| TEXAS INSTRUMENTS INCORPORATED
| Standard Linear and Logic Group
| IBIS Model of SN74ALVCH162827
| 20-BIT BUFFER/DRIVER WITH 3-STATE OUTPUTS
| This file contains package information for the following:
|  TSSOP 56-pin (DGG) package as [Component] ALVCH162827_DGG
|  TVSOP 56-pin (DGV) package as [Component] ALVCH162827_DGV
|  SSOP 56-pin (DL) package as [Component] ALVCH162827_DL
| This device can be powered at the following Vccs:
|  1.8 volt Vcc
|  2.5 volt Vcc
|  2.7 volt Vcc
|  3.3 volt Vcc
| This file provides unique models under the [Model Selector] for each Vcc.
| For operation at a specific Vcc, select the appropriate model after each
| [Model Selector] keyword.
[IBIS Ver]   3.2
[Comment char]  |_char
[File Name]   sn74alvch162827.ibs
[File Rev]   1.1 | a_die
[Date]   May 5, 2003
[Source]   Data created from TI-SPICE simulations at TI-SLL.
[Notes]   The following is an IBIS list for the ALVCH162827.
   Please contact sllibis@ti.com with questions and
   comments concerning SLL IBIS models.
   This IBIS model is created from a BA (back annotated
   netlist)
   - Non-monotonic data in ground-clamp due to bus-hold
[Disclaimer] Property of Texas Instruments Incorporated.  Unauthorized
   reproduction and/or distribution is strictly prohibited.
   This product is protected under copyright law.
   Created  2003, (C) Copyright  2003, Texas Instruments
   Incorporated, All Rights Reserved
   UNLESS THERE IS A SIGNED, WRITTEN AGREEMENT TO THE
   CONTRARY, TEXAS INSTRUMENTS (TI) IS PROVIDING THE IBIS
   MODELS  AND WITHOUT ANY WARRANTY, EXPRESSED OR
   IMPLIED.  TI assumes no liability for:
   1) the accuracy of the IBIS models provided to your
   company;
   2) the proper functioning of these IBIS Models in your
   design or for any resulting applications; or
   3) infringement of patents, copyrights or intellectual
   property rights resulting from your use of these IBIS
   models.
   TI provides IBIS Models as a service to our customers.
   You and your company shall not distribute, sell or give
   these models to anyone else without prior written
   permission from TI.
   TI reserves the right to make changes to our products or
   to discontinue any semiconductor product or service
   without notice, and advises our customers to obtain the
   latest version of relevant information to verify, before
   placing orders, that the information being relied on is
   current.
   Please be aware that your receipt and use of the IBIS
   information provided shall serve as acceptance of these
   terms and conditions.  If you do not accept these terms,
   you should return or destroy the IBIS models and any
   other accompanying information immediately.
| Component ALVCH162827_DGG 56-pin TSSOP
[Component]   ALVCH162827_DGG
[Manufacturer]   Texas Instruments, Inc.
[Package]
|   typ   min   max
R_pkg   4.500e-02   3.500e-02   6.200e-02
L_pkg   3.324e-09   2.403e-09   5.094e-09
C_pkg   5.640e-13   3.410e-13   9.140e-13
[Pin]   signal_name   model_name   R_pin   L_pin   C_pin
1   1NOE1   ALVCH162827_OE   6.200e-02   5.094e-09   8.560e-13
2   1Y1   ALVCH162827_OUT   6.100e-02   4.621e-09   9.020e-13
3   1Y2   ALVCH162827_OUT   6.000e-02   4.316e-09   8.020e-13
4   GND   GND   5.900e-02   3.968e-09   6.980e-13
5   1Y3   ALVCH162827_OUT   5.700e-02   3.716e-09   6.490e-13
6   1Y4   ALVCH162827_OUT   4.200e-02   3.517e-09   6.530e-13
7   VCC   POWER   4.100e-02   3.160e-09   5.700e-13
8   1Y5   ALVCH162827_OUT   3.900e-02   2.981e-09   4.820e-13
9   1Y6   ALVCH162827_OUT   3.900e-02   2.808e-09   4.470e-13
10   1Y7   ALVCH162827_OUT   3.800e-02   2.715e-09   4.090e-13
11   GND   GND   4.100e-02   2.675e-09   3.910e-13
12   1Y8   ALVCH162827_OUT   3.900e-02   2.536e-09   3.660e-13
13   1Y9   ALVCH162827_OUT   3.900e-02   2.457e-09   3.480e-13
14   1Y10   ALVCH162827_OUT   3.800e-02   2.411e-09   3.530e-13
15   2Y1   ALVCH162827_OUT   3.900e-02   2.456e-09   3.550e-13
16   2Y2   ALVCH162827_OUT   3.900e-02   2.471e-09   3.490e-13
17   2Y3   ALVCH162827_OUT   4.000e-02   2.580e-09   3.700e-13
18   GND   GND   3.800e-02   2.651e-09   3.890e-13
19   2Y4   ALVCH162827_OUT   3.800e-02   2.739e-09   4.110e-13
20   2Y5   ALVCH162827_OUT   3.900e-02   2.838e-09   4.490e-13
21   2Y6   ALVCH162827_OUT   3.800e-02   2.988e-09   4.840e-13
22   VCC   POWER   3.800e-02   3.104e-09   5.640e-13
23   2Y7   ALVCH162827_OUT   4.000e-02   3.427e-09   6.380e-13
24   2Y8   ALVCH162827_OUT   5.600e-02   3.654e-09   6.410e-13
25   GND   GND   5.700e-02   3.932e-09   7.000e-13
26   2Y9   ALVCH162827_OUT   5.800e-02   4.257e-09   8.060e-13
27   2Y10   ALVCH162827_OUT   5.700e-02   4.580e-09   9.140e-13
28   2NOE1   ALVCH162827_OE   5.900e-02   5.038e-09   8.610e-13
29   2NOE2   ALVCH162827_OE   6.000e-02   5.058e-09   8.580e-13
30   2A10   ALVCH162827_IN   5.600e-02   4.543e-09   9.040e-13
31   2A9   ALVCH162827_IN   5.700e-02   4.241e-09   8.020e-13
32   GND   GND   5.900e-02   3.933e-09   6.990e-13
33   2A8   ALVCH162827_IN   5.600e-02   3.616e-09   6.370e-13
34   2A7   ALVCH162827_IN   3.700e-02   3.368e-09   6.400e-13
35   VCC   POWER   3.600e-02   3.024e-09   5.630e-13
36   2A6   ALVCH162827_IN   3.500e-02   2.876e-09   4.740e-13
37   2A5   ALVCH162827_IN   3.500e-02   2.745e-09   4.440e-13
38   2A4   ALVCH162827_IN   3.700e-02   2.683e-09   4.050e-13
39   GND   GND   3.800e-02   2.603e-09   3.820e-13
40   2A3   ALVCH162827_IN   3.800e-02   2.510e-09   3.620e-13
41   2A2   ALVCH162827_IN   3.600e-02   2.412e-09   3.410e-13
42   2A1   ALVCH162827_IN   3.800e-02   2.416e-09   3.490e-13
43   1A10   ALVCH162827_IN   3.800e-02   2.403e-09   3.490e-13
44   1A9   ALVCH162827_IN   3.700e-02   2.429e-09   3.410e-13
45   1A8   ALVCH162827_IN   3.600e-02   2.483e-09   3.580e-13
46   GND   GND   3.700e-02   2.614e-09   3.810e-13
47   1A7   ALVCH162827_IN   3.500e-02   2.669e-09   4.020e-13
48   1A6   ALVCH162827_IN   3.600e-02   2.763e-09   4.420e-13
49   1A5   ALVCH162827_IN   3.600e-02   2.942e-09   4.780e-13
50   VCC   POWER   3.500e-02   3.053e-09   5.640e-13
51   1A4   ALVCH162827_IN   3.600e-02   3.408e-09   6.410e-13
52   1A3   ALVCH162827_IN   5.800e-02   3.698e-09   6.410e-13
53   GND   GND   5.900e-02   3.974e-09   6.970e-13
54   1A2   ALVCH162827_IN   6.100e-02   4.327e-09   8.020e-13
55   1A1   ALVCH162827_IN   6.100e-02   4.624e-09   9.050e-13
56   1NOE2   ALVCH162827_OE   6.000e-02   5.063e-09   8.580e-13
| Component ALVCH162827_DGV 56-pin TVSOP
[Component]   ALVCH162827_DGV
[Manufacturer]   Texas Instruments, Inc.
[Package]
|   typ   min   max
R_pkg   6.300e-02   5.000e-02   8.400e-02
L_pkg   2.945e-09   2.394e-09   3.939e-09
C_pkg   3.910e-13   2.710e-13   5.880e-13
[Pin]   signal_name   model_name   R_pin   L_pin   C_pin
1   1NOE1   ALVCH162827_OE   6.800e-02   3.933e-09   5.880e-13
2   1Y1   ALVCH162827_OUT   6.800e-02   3.568e-09   5.870e-13
3   1Y2   ALVCH162827_OUT   7.600e-02   3.464e-09   5.150e-13
4   GND   GND   8.400e-02   3.444e-09   4.590e-13
5   1Y3   ALVCH162827_OUT   8.100e-02   3.277e-09   4.270e-13
6   1Y4   ALVCH162827_OUT   7.400e-02   3.136e-09   3.870e-13
7   VCC   POWER   6.900e-02   2.970e-09   4.010e-13
8   1Y5   ALVCH162827_OUT   5.000e-02   2.785e-09   3.790e-13
9   1Y6   ALVCH162827_OUT   5.100e-02   2.685e-09   3.200e-13
10   1Y7   ALVCH162827_OUT   5.300e-02   2.611e-09   3.160e-13
11   GND   GND   5.300e-02   2.495e-09   2.970e-13
12   1Y8   ALVCH162827_OUT   5.300e-02   2.435e-09   2.920e-13
13   1Y9   ALVCH162827_OUT   5.500e-02   2.412e-09   2.850e-13
14   1Y10   ALVCH162827_OUT   5.600e-02   2.401e-09   2.730e-13
15   2Y1   ALVCH162827_OUT   5.500e-02   2.401e-09   2.730e-13
16   2Y2   ALVCH162827_OUT   5.500e-02   2.399e-09   2.840e-13
17   2Y3   ALVCH162827_OUT   5.400e-02   2.406e-09   2.890e-13
18   GND   GND   5.300e-02   2.450e-09   2.930e-13
19   2Y4   ALVCH162827_OUT   5.100e-02   2.544e-09   3.110e-13
20   2Y5   ALVCH162827_OUT   5.100e-02   2.626e-09   3.150e-13
21   2Y6   ALVCH162827_OUT   5.000e-02   2.727e-09   3.690e-13
22   VCC   POWER   6.500e-02   2.903e-09   3.930e-13
23   2Y7   ALVCH162827_OUT   7.500e-02   3.091e-09   3.860e-13
24   2Y8   ALVCH162827_OUT   8.200e-02   3.272e-09   4.280e-13
25   GND   GND   8.200e-02   3.393e-09   4.570e-13
26   2Y9   ALVCH162827_OUT   7.300e-02   3.380e-09   5.080e-13
27   2Y10   ALVCH162827_OUT   7.100e-02   3.577e-09   5.800e-13
28   2NOE1   ALVCH162827_OE   6.800e-02   3.937e-09   5.740e-13
29   2NOE2   ALVCH162827_OE   6.900e-02   3.923e-09   5.690e-13
30   2A10   ALVCH162827_IN   6.400e-02   3.536e-09   5.740e-13
31   2A9   ALVCH162827_IN   7.600e-02   3.428e-09   5.170e-13
32   GND   GND   8.100e-02   3.395e-09   4.680e-13
33   2A8   ALVCH162827_IN   8.000e-02   3.255e-09   4.310e-13
34   2A7   ALVCH162827_IN   7.100e-02   3.064e-09   3.860e-13
35   VCC   POWER   6.100e-02   2.878e-09   3.890e-13
36   2A6   ALVCH162827_IN   5.000e-02   2.710e-09   3.630e-13
37   2A5   ALVCH162827_IN   5.000e-02   2.606e-09   3.110e-13
38   2A4   ALVCH162827_IN   5.200e-02   2.534e-09   3.060e-13
39   GND   GND   5.200e-02   2.439e-09   2.890e-13
40   2A3   ALVCH162827_IN   5.300e-02   2.399e-09   2.860e-13
41   2A2   ALVCH162827_IN   5.500e-02   2.394e-09   2.820e-13
42   2A1   ALVCH162827_IN   5.500e-02   2.398e-09   2.710e-13
43   1A10   ALVCH162827_IN   5.600e-02   2.396e-09   2.710e-13
44   1A9   ALVCH162827_IN   5.400e-02   2.402e-09   2.830e-13
45   1A8   ALVCH162827_IN   5.400e-02   2.423e-09   2.880e-13
46   GND   GND   5.300e-02   2.474e-09   2.920e-13
47   1A7   ALVCH162827_IN   5.100e-02   2.569e-09   3.090e-13
48   1A6   ALVCH162827_IN   5.100e-02   2.638e-09   3.130e-13
49   1A5   ALVCH162827_IN   5.100e-02   2.742e-09   3.660e-13
50   VCC   POWER   6.400e-02   2.917e-09   3.900e-13
51   1A4   ALVCH162827_IN   7.400e-02   3.083e-09   3.830e-13
52   1A3   ALVCH162827_IN   8.100e-02   3.249e-09   4.300e-13
53   GND   GND   8.300e-02   3.400e-09   4.550e-13
54   1A2   ALVCH162827_IN   7.500e-02   3.427e-09   5.050e-13
55   1A1   ALVCH162827_IN   7.100e-02   3.585e-09   5.780e-13
56   1NOE2   ALVCH162827_OE   6.900e-02   3.939e-09   5.810e-13
| Component ALVCH162827_DL 56-pin SSOP
[Component]   ALVCH162827_DL
[Manufacturer]   Texas Instruments, Inc.
[Package]
|   typ   min   max
R_pkg   5.500e-02   4.800e-02   6.700e-02
L_pkg   6.539e-09   4.803e-09   9.746e-09
C_pkg   8.570e-13   5.000e-13   1.351e-12
[Pin]   signal_name   model_name   R_pin   L_pin   C_pin
1   1NOE1   ALVCH162827_OE   6.400e-02   9.646e-09   1.202e-12
2   1Y1   ALVCH162827_OUT   5.900e-02   8.723e-09   1.348e-12
3   1Y2   ALVCH162827_OUT   5.900e-02   8.139e-09   1.223e-12
4   GND   GND   5.600e-02   7.554e-09   1.088e-12
5   1Y3   ALVCH162827_OUT   5.400e-02   6.991e-09   9.660e-13
6   1Y4   ALVCH162827_OUT   5.300e-02   6.659e-09   9.730e-13
7   VCC   POWER   5.500e-02   6.321e-09   9.050e-13
8   1Y5   ALVCH162827_OUT   5.600e-02   5.942e-09   7.130e-13
9   1Y6   ALVCH162827_OUT   5.700e-02   5.768e-09   6.780e-13
10   1Y7   ALVCH162827_OUT   5.400e-02   5.459e-09   6.310e-13
11   GND   GND   5.100e-02   5.224e-09   6.380e-13
12   1Y8   ALVCH162827_OUT   4.800e-02   5.088e-09   6.010e-13
13   1Y9   ALVCH162827_OUT   5.000e-02   5.021e-09   5.180e-13
14   1Y10   ALVCH162827_OUT   5.100e-02   4.803e-09   5.000e-13
15   2Y1   ALVCH162827_OUT   5.100e-02   4.803e-09   5.000e-13
16   2Y2   ALVCH162827_OUT   5.000e-02   5.021e-09   5.180e-13
17   2Y3   ALVCH162827_OUT   4.800e-02   5.088e-09   6.010e-13
18   GND   GND   5.100e-02   5.224e-09   6.380e-13
19   2Y4   ALVCH162827_OUT   5.400e-02   5.459e-09   6.310e-13
20   2Y5   ALVCH162827_OUT   5.700e-02   5.768e-09   6.770e-13
21   2Y6   ALVCH162827_OUT   5.500e-02   5.942e-09   7.150e-13
22   VCC   POWER   5.500e-02   6.321e-09   9.070e-13
23   2Y7   ALVCH162827_OUT   5.300e-02   6.659e-09   9.720e-13
24   2Y8   ALVCH162827_OUT   5.400e-02   6.991e-09   9.660e-13
25   GND   GND   5.600e-02   7.554e-09   1.087e-12
26   2Y9   ALVCH162827_OUT   5.900e-02   8.139e-09   1.223e-12
27   2Y10   ALVCH162827_OUT   5.900e-02   8.727e-09   1.351e-12
28   2NOE1   ALVCH162827_OE   6.700e-02   9.746e-09   1.210e-12
29   2NOE2   ALVCH162827_OE   6.300e-02   9.630e-09   1.203e-12
30   2A10   ALVCH162827_IN   6.000e-02   8.751e-09   1.349e-12
31   2A9   ALVCH162827_IN   6.000e-02   8.184e-09   1.224e-12
32   GND   GND   5.600e-02   7.543e-09   1.087e-12
33   2A8   ALVCH162827_IN   5.400e-02   7.005e-09   9.690e-13
34   2A7   ALVCH162827_IN   5.600e-02   6.714e-09   9.750e-13
35   VCC   POWER   5.800e-02   6.384e-09   9.090e-13
36   2A6   ALVCH162827_IN   5.700e-02   5.976e-09   7.170e-13
37   2A5   ALVCH162827_IN   5.700e-02   5.743e-09   6.770e-13
38   2A4   ALVCH162827_IN   5.400e-02   5.468e-09   6.310e-13
39   GND   GND   5.500e-02   5.329e-09   6.440e-13
40   2A3   ALVCH162827_IN   5.200e-02   5.189e-09   6.060e-13
41   2A2   ALVCH162827_IN   5.200e-02   5.053e-09   5.190e-13
42   2A1   ALVCH162827_IN   5.200e-02   4.825e-09   5.020e-13
43   1A10   ALVCH162827_IN   5.400e-02   4.897e-09   5.060e-13
44   1A9   ALVCH162827_IN   5.200e-02   5.093e-09   5.210e-13
45   1A8   ALVCH162827_IN   5.100e-02   5.179e-09   6.080e-13
46   GND   GND   5.400e-02   5.314e-09   6.450e-13
47   1A7   ALVCH162827_IN   5.500e-02   5.511e-09   6.320e-13
48   1A6   ALVCH162827_IN   5.700e-02   5.770e-09   6.770e-13
49   1A5   ALVCH162827_IN   5.600e-02   5.956e-09   7.160e-13
50   VCC   POWER   5.500e-02   6.320e-09   9.050e-13
51   1A4   ALVCH162827_IN   5.200e-02   6.621e-09   9.680e-13
52   1A3   ALVCH162827_IN   5.300e-02   6.974e-09   9.660e-13
53   GND   GND   5.700e-02   7.571e-09   1.089e-12
54   1A2   ALVCH162827_IN   5.700e-02   8.097e-09   1.219e-12
55   1A1   ALVCH162827_IN   5.900e-02   8.723e-09   1.349e-12
56   1NOE2   ALVCH162827_OE   6.100e-02   9.560e-09   1.199e-12
| Model ALVCH162827_IN
[Model Selector]   ALVCH162827_IN
ALVCH162827_IN_18   1.8 volt Vcc
ALVCH162827_IN_25   2.5 volt Vcc
ALVCH162827_IN_33   3.3 volt Vcc
| Model ALVCH162827_OE
[Model Selector]   ALVCH162827_OE
ALVCH162827_OE_18   1.8 volt Vcc
ALVCH162827_OE_25   2.5 volt Vcc
ALVCH162827_OE_33   3.3 volt Vcc
| Model ALVCH162827_OUT
[Model Selector]   ALVCH162827_OUT
ALVCH162827_OUT_18   1.8 volt Vcc
ALVCH162827_OUT_25   2.5 volt Vcc
ALVCH162827_OUT_33   3.3 volt Vcc
| Models and submodels in the file (9): ALVCH162827_IN_18 (Input), ALVCH162827_IN_25 (Input), ALVCH162827_IN_33 (Input), ALVCH162827_OE_18 (Input), ALVCH162827_OE_25 (Input), ALVCH162827_OE_33 (Input), ALVCH162827_OUT_18 (3-state), ALVCH162827_OUT_25 (3-state), ALVCH162827_OUT_33 (3-state)
